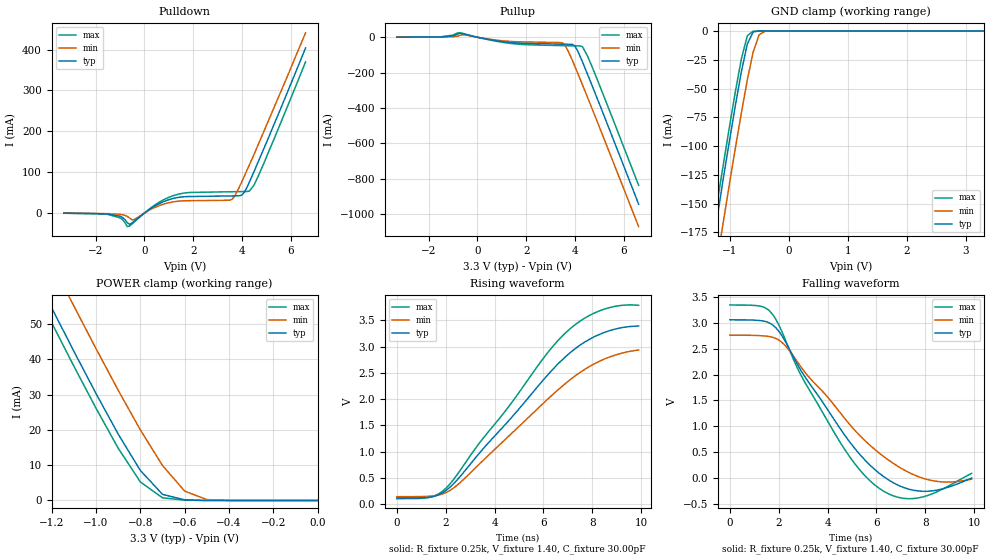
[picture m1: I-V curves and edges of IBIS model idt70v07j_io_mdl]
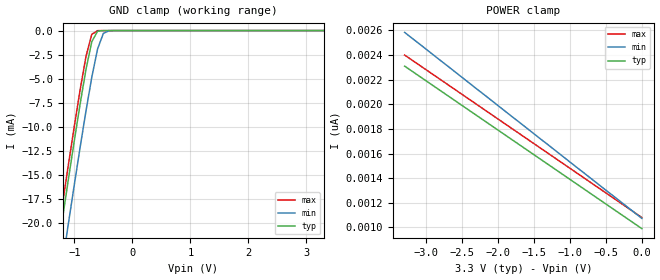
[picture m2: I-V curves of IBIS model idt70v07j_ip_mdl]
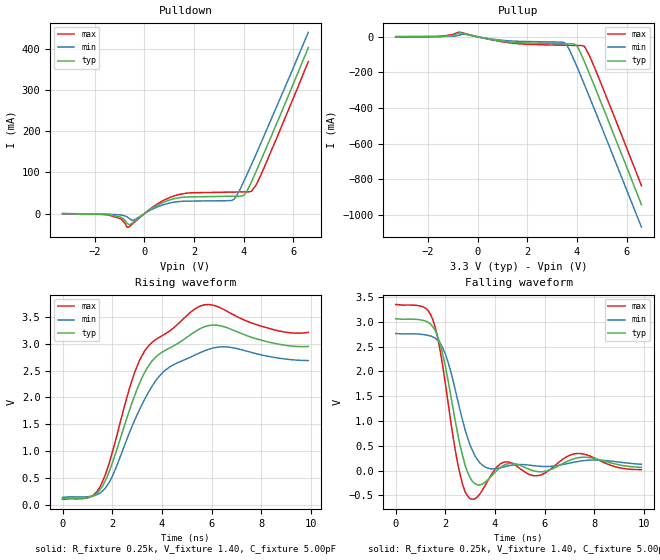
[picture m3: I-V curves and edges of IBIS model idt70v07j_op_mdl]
| IBIS file 70v07j.ibs created by s2ibis2 version 1.0
| North Carolina State University Electronics Research Laboratory  1995
[IBIS ver]   2.1
[File name]   70v07j.ibs
[File Rev]   3.1
[Date]   06/18/97
[Source]   Integrated Device Technology, Inc.
[Notes]   1.Temperatures: typ=25C, min=100C, max=0C 2.Cemos7_5v process.
   3.RRmp rates based on 50 ohm load.
[Disclaimer]   This information is for modeling purpose only, and is not
   guaranteed.
[Copyright]   Copyright 1997, Integrated Device Technology, Inc. all rights
   reserved
|   Component idt70v07j
[Component]   idt70v07j
[Manufacturer]   Integrated Device Technology
[Package]
| variable   typ   min   max
R_pkg   100.00m   50.00m   0.15
L_pkg   12.00nH   11.00nH   13.00nH
C_pkg   0.80pF   0.70pF   0.90pF
[Pin]  signal_name   model_name   R_pin   L_pin   C_pin
1   A13L   idt70v07j_ip_mdl
2   A14L   idt70v07j_ip_mdl
3   CEBL   idt70v07j_ip_mdl
4   SEMBL   idt70v07j_ip_mdl
5   RWBL   idt70v07j_ip_mdl
6   OEBL   idt70v07j_ip_mdl
7   NC   NC
8   IO0L   idt70v07j_io_mdl
9   IO1L   idt70v07j_io_mdl
10   IO2L   idt70v07j_io_mdl
11   IO3L   idt70v07j_io_mdl
12   IO4L   idt70v07j_io_mdl
13   IO5L   idt70v07j_io_mdl
14   GND   GND
15   IO6L   idt70v07j_io_mdl
16   IO7L   idt70v07j_io_mdl
17   VCC   POWER
18   GND   GND
19   IO0R   idt70v07j_io_mdl
20   IO1R   idt70v07j_io_mdl
21   IO2R   idt70v07j_io_mdl
22   VCC   POWER
23   IO3R   idt70v07j_io_mdl
24   IO4R   idt70v07j_io_mdl
25   IO5R   idt70v07j_io_mdl
26   IO6R   idt70v07j_io_mdl
27   IO7R   idt70v07j_io_mdl
28   NC   NC
29   OEBR   idt70v07j_ip_mdl
30   RWBR   idt70v07j_ip_mdl
31   SEMBR   idt70v07j_ip_mdl
32   CEBR   idt70v07j_ip_mdl
33   A14R   idt70v07j_ip_mdl
34   A13R   idt70v07j_ip_mdl
35   GND   GND
36   A12R   idt70v07j_ip_mdl
37   A11R   idt70v07j_ip_mdl
38   A10R   idt70v07j_ip_mdl
39   A9R   idt70v07j_ip_mdl
40   A8R   idt70v07j_ip_mdl
41   A7R   idt70v07j_ip_mdl
42   A6R   idt70v07j_ip_mdl
43   A5R   idt70v07j_ip_mdl
44   A4R   idt70v07j_ip_mdl
45   A3R   idt70v07j_ip_mdl
46   A2R   idt70v07j_ip_mdl
47   A1R   idt70v07j_ip_mdl
48   A0R   idt70v07j_ip_mdl
49   INTBR   idt70v07j_io_mdl
50   BUSYBR   idt70v07j_io_mdl
51   MSB   idt70v07j_ip_mdl
52   GND   GND
53   BUSYBL   idt70v07j_io_mdl
54   INTBL   idt70v07j_io_mdl
55   A0L   idt70v07j_ip_mdl
56   A1L   idt70v07j_ip_mdl
57   A2L   idt70v07j_ip_mdl
58   A3L   idt70v07j_ip_mdl
59   A4L   idt70v07j_ip_mdl
60   A5L   idt70v07j_ip_mdl
61   A6L   idt70v07j_ip_mdl
62   A7L   idt70v07j_ip_mdl
63   A8L   idt70v07j_ip_mdl
64   A9L   idt70v07j_ip_mdl
65   A10L   idt70v07j_ip_mdl
66   A11L   idt70v07j_ip_mdl
67   A12L   idt70v07j_ip_mdl
68   VCC   POWER
| Models and submodels in the file (3): idt70v07j_io_mdl (I/O), idt70v07j_ip_mdl (Input), idt70v07j_op_mdl (Output)
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| in1  in1   dummy_model
| oel1 oel1   dummy_model
| in2  in2   dummy_model
| oel2 oel2   dummy_model
|   Model idt70v07j_io_mdl
[Model]   idt70v07j_io_mdl
Model_type   I/O
Polarity   Non-Inverting
Enable   Active-High
Vinl =  0.800V
Vinh =  2.200V
Vmeas =  1.500V
C_comp   3.00pF   NA   NA
[Temperature Range]   25.00   100.00   0.000
[Voltage Range]   3.30V   3.00V   3.60V
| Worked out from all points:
|   slope of the pulldown table from 0 to 0.495 V, typ, clamps not added: 25.2 ohm
|   slope of the pullup table from 0 to 0.495 V, typ, clamps not added: 36.8 ohm
|   GND clamp passes 1 mA (typ) near -0.60 V on its own axis
|   POWER clamp passes 1 mA (typ) near -0.65 V on its own axis
|   rising waveform, R_fixture 0.25k, V_fixture 1.40, C_fixture 30.00pF: 20-80 % time 3.72ns typ, 3.88ns min, 3.59ns max; typ from 0.115 V to 3.39 V
|   falling waveform, R_fixture 0.25k, V_fixture 1.40, C_fixture 30.00pF: 20-80 % time 2.56ns typ, 3.15ns min, 2.2ns max; typ from 3.06 V to -0.003 V
[Pulldown]
| voltage   I(typ)   I(min)   I(max)
-3.3V     -100uA     100uA      -300uA
-1.5V     -2.3mA     -1.4mA     -3.1mA
-1V       -7.58mA    -3.1mA     -11.52mA
-700mV    -23.57mA   -8.02mA    -32.97mA
-400mV    -18.78mA   -15.14mA   -20.95mA
400mV     16.4mA     13.1mA     18.68mA
1.2V      36.14mA    27.71mA    42.98mA
3.6V      42.09mA    34.37mA    52.29mA
4V        44.32mA    78.11mA    52.68mA
4.3V      75.97mA    118mA      53.81mA
4.5V      103mA      145mA      69.61mA
6.6V      404mA      441mA      370mA
[Pullup]
| voltage   I(typ)   I(min)   I(max)
-3.3V     600uA      600uA      600uA
-1.5V     1.72mA     1.3mA      2.05mA
-1V       7.22mA     2.99mA     12.15mA
-700mV    21.94mA    10.89mA    24.98mA
1.3V      -29.2mA    -23.2mA    -33.88mA
3.5V      -39.14mA   -33.41mA   -47.46mA
3.7V      -39.55mA   -74.44mA   -47.96mA
3.9V      -40.72mA   -135mA     -48.42mA
4V        -51.77mA   -168mA     -48.63mA
4.3V      -139mA     -269mA     -53.53mA
4.5V      -207mA     -337mA     -104mA
6.6V      -944mA     -1.071A    -837mA
[GND_clamp]
| voltage   I(typ)   I(min)   I(max)
-3.3V     -864mA     -899mA     -853mA
-1.3V     -191mA     -229mA     -179mA
-1.2V     -159mA     -196mA     -146mA
-1.1V     -126mA     -164mA     -114mA
-1V       -94.82mA   -132mA     -82.47mA
-900mV    -64.06mA   -101mA     -51.97mA
-800mV    -35.17mA   -70.9mA    -24.01mA
-700mV    -11.19mA   -42.49mA   -4.125mA
-600mV    -762uA     -18.03mA   -100uA
-500mV    -17.07uA   -3.206mA   -1.452uA
-400mV    -350nA     -181uA     -22.4nA
3.3V      3.959nA    390nA      3.869nA
[POWER_clamp]
| voltage   I(typ)   I(min)   I(max)
-3.3V     325mA      337mA      321mA
-1.3V     67.04mA    79.86mA    62.82mA
-1.2V     54.58mA    67.42mA    50.35mA
-1.1V     42.29mA    55.12mA    38.07mA
-1V       30.3mA     43.02mA    26.13mA
-900mV    18.81mA    31.24mA    14.82mA
-800mV    8.514mA    20mA       5.253mA
-700mV    1.731mA    9.91mA     761uA
-600mV    187uA      2.654mA    85.3uA
-500mV    802nA      257uA      72.72nA
-400mV    20.83nA    8.596uA    5.886nA
0V        3.959nA    5.788nA    4.32nA
[Ramp]
| variable   typ   min   max
dV/dt_r   0.94/3.55n   0.73/3.56n   1.12/3.50n
dV/dt_f   1.12/3.31n   0.86/3.52n   1.34/3.07n
R_load = 50.00
[Rising Waveform]
R_fixture = 0.25k
V_fixture = 1.40
C_fixture = 30.00pF
R_dut = 100.00m
L_dut = 12.00nH
C_dut = 0.80pF
| time   V(typ)   V(min)   V(max)
0s        115mV      140mV      103mV
1.4ns     137mV      152mV      134mV
2ns       257mV      217mV      298mV
2.7ns     585mV      456mV      714mV
6.1ns     2.42V      1.965V     2.839V
7.2ns     2.923V     2.407V     3.381V
7.8ns     3.116V     2.597V     3.572V
8.5ns     3.271V     2.764V     3.716V
9.2ns     3.361V     2.874V     3.786V
9.9ns     3.393V     2.936V     3.788V
[Falling Waveform]
R_fixture = 0.25k
V_fixture = 1.40
C_fixture = 30.00pF
R_dut = 100.00m
L_dut = 12.00nH
C_dut = 0.80pF
| time   V(typ)   V(min)   V(max)
0s        3.063V     2.766V     3.351V
1.3ns     3.044V     2.754V     3.32V
1.8ns     2.944V     2.716V     3.136V
2.9ns     2.088V     2.157V     1.998V
4.5ns     965mV      1.273V     701mV
5.3ns     465mV      831mV      165mV
6.1ns     95.66mV    487mV      -197mV
6.9ns     -144mV     218mV      -378mV
7.7ns     -253mV     27.95mV    -389mV
9.9ns     -3.257mV   -24.68mV   87.7mV
|   Model idt70v07j_ip_mdl
[Model]   idt70v07j_ip_mdl
Model_type   Input
Vinl =  0.800V
Vinh =  2.200V
Vmeas =  1.500V
C_comp   3.00pF   NA   NA
[Temperature Range]   25.00   100.00   0.000
[Voltage Range]   3.30V   3.00V   3.60V
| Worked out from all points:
|   GND clamp passes 1 mA (typ) near -0.69 V on its own axis
[GND_clamp]
| voltage   I(typ)   I(min)   I(max)
-3.3V     -107mA     -111mA     -106mA
-1.3V     -23.44mA   -28.04mA   -21.93mA
-1.2V     -19.38mA   -23.99mA   -17.87mA
-1.1V     -15.37mA   -19.98mA   -13.85mA
-1V       -11.43mA   -16.02mA   -9.925mA
-900mV    -7.614mA   -12.13mA   -6.142mA
-800mV    -4.046mA   -8.382mA   -2.703mA
-700mV    -1.162mA   -4.871mA   -391uA
-600mV    -66.77uA   -1.916mA   -7.976uA
-500mV    -1.353uA   -291uA     -115nA
-400mV    -28.11nA   -14.45uA   -2.16nA
3.3V      990pA      1.211nA    960pA
[POWER_clamp]
| voltage   I(typ)   I(min)   I(max)
-3.3V     2.31nA     2.584nA    2.4nA
-900mV    1.35nA     1.485nA    1.44nA
-400mV    1.15nA     1.257nA    1.24nA
0V        990pA      1.073nA    1.08nA
|   Model idt70v07j_op_mdl
[Model]   idt70v07j_op_mdl
Model_type   Output
Polarity   Non-Inverting
Enable   Active-High
Vinl =  0.800V
Vinh =  2.200V
Vmeas =  1.500V
C_comp   3.00pF   NA   NA
[Temperature Range]   25.00   100.00   0.000
[Voltage Range]   3.30V   3.00V   3.60V
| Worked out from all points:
|   slope of the pulldown table from 0 to 0.495 V, typ, clamps not added: 25.2 ohm
|   slope of the pullup table from 0 to 0.495 V, typ, clamps not added: 36.8 ohm
|   rising waveform, R_fixture 0.25k, V_fixture 1.40, C_fixture 5.00pF: 20-80 % time 1.29ns typ, 1.45ns min, 1.17ns max; typ from 0.115 V to 2.95 V
|   falling waveform, R_fixture 0.25k, V_fixture 1.40, C_fixture 5.00pF: 20-80 % time 692ps typ, 827ps min, 620ps max; typ from 3.06 V to 0.066 V
[Pulldown]
| voltage   I(typ)   I(min)   I(max)
-3.3V     -200uA     100uA      -300uA
-1.5V     -2.3mA     -1.4mA     -3mA
-1V       -7.56mA    -3.1mA     -11.52mA
-700mV    -23.67mA   -8.02mA    -33.09mA
-400mV    -18.78mA   -15.15mA   -20.95mA
400mV     16.4mA     13.1mA     18.68mA
1.2V      36.14mA    27.71mA    42.98mA
3.6V      42.09mA    34.37mA    52.29mA
4V        44.32mA    78.11mA    52.68mA
4.3V      75.97mA    118mA      53.81mA
4.5V      103mA      145mA      69.61mA
6.6V      404mA      441mA      370mA
[Pullup]
| voltage   I(typ)   I(min)   I(max)
-3.3V     600uA      500uA      600uA
-1.5V     1.72mA     1.3mA      2.05mA
-1V       7.22mA     2.99mA     12.15mA
-700mV    21.94mA    10.89mA    24.98mA
1.3V      -29.2mA    -23.2mA    -33.88mA
3.5V      -39.14mA   -33.27mA   -47.46mA
3.7V      -39.55mA   -74.07mA   -47.96mA
3.9V      -40.67mA   -135mA     -48.42mA
4V        -51.55mA   -167mA     -48.63mA
4.3V      -139mA     -268mA     -53.38mA
4.5V      -206mA     -336mA     -104mA
6.6V      -942mA     -1.068A    -835mA
[Ramp]
| variable   typ   min   max
dV/dt_r   0.94/3.56n   0.73/3.57n   1.12/3.51n
dV/dt_f   1.12/3.32n   0.86/3.52n   1.34/3.08n
R_load = 50.00
[Rising Waveform]
R_fixture = 0.25k
V_fixture = 1.40
C_fixture = 5.00pF
R_dut = 100.00m
L_dut = 12.00nH
C_dut = 0.80pF
| time   V(typ)   V(min)   V(max)
0s        115mV      140mV      103mV
1.4ns     220mV      193mV      258mV
2ns       770mV      529mV      972mV
2.7ns     1.769V     1.352V     2.178V
3.2ns     2.369V     1.868V     2.777V
4.1ns     2.868V     2.493V     3.174V
5.3ns     3.214V     2.783V     3.639V
6.6ns     3.303V     2.941V     3.611V
8.4ns     3.021V     2.756V     3.275V
9.9ns     2.95V      2.687V     3.211V
[Falling Waveform]
R_fixture = 0.25k
V_fixture = 1.40
C_fixture = 5.00pF
R_dut = 100.00m
L_dut = 12.00nH
C_dut = 0.80pF
| time   V(typ)   V(min)   V(max)
0s        3.063V     2.766V     3.351V
1.5ns     2.896V     2.697V     3.041V
2ns       2.113V     2.357V     1.753V
2.5ns     741mV      1.413V     135mV
3ns       -144mV     511mV      -568mV
3.6ns     -234mV     71.27mV    -302mV
4.4ns     118mV      80.03mV    174mV
5.7ns     -19.22mV   92.75mV    -102mV
7.4ns     264mV      190mV      346mV
9.9ns     65.88mV    128mV      19.45mV
